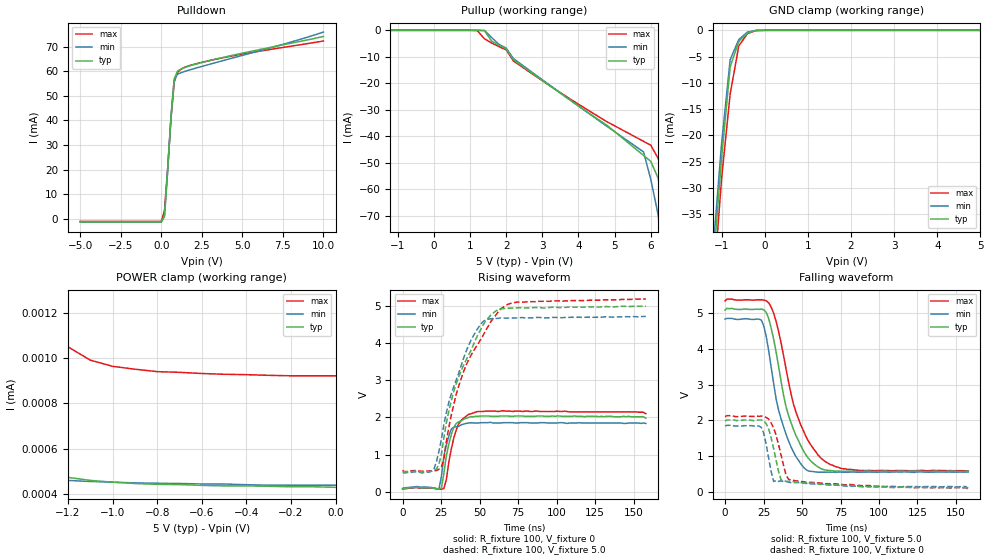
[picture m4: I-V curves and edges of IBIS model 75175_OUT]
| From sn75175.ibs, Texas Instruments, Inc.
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|   Model 75175_OUT
[Model]   75175_OUT
Model_type  3-state
Polarity   Non-Inverting
Enable   Active-Low
Vmeas = 1.3V
Cref = 15pf
Vref = 0V
| variable   typ   min   max
C_comp   3.716pf   3.575pf   4.006pf
[Temperature Range]   25   0   70
[Voltage Range]   5.0   4.75   5.25
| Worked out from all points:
|   slope of the pulldown table from 0 to 0.75 V, typ, clamps not added: 13.8 ohm
|   GND clamp passes 1 mA (typ) near -0.46 V on its own axis
|   rising waveform, R_fixture 100, V_fixture 0: 20-80 % time 5.45ns typ, 4.65ns min, 6.22ns max; typ from 0.094 V to 1.98 V
|   falling waveform, R_fixture 100, V_fixture 5.0: 20-80 % time 15.1ns typ, 13.2ns min, 17.4ns max; typ from 5.08 V to 0.587 V
|   rising waveform, R_fixture 100, V_fixture 5.0: 20-80 % time 20.8ns typ, 17.3ns min, 24ns max; typ from 0.548 V to 4.99 V
|   falling waveform, R_fixture 100, V_fixture 0: 20-80 % time 6.07ns typ, 4.76ns min, 7.27ns max; typ from 1.98 V to 0.096 V
[Pulldown]
|   Voltage   I(typ)   I(min   I(max)
-5V       -1.312mA   -1.5mA     -1.165mA
0V        -1.312mA   -1.5mA     -1.165mA
200mV     1.139mA    857.1uA    3.313mA
400mV     20.56mA    19.69mA    20.96mA
600mV     41.35mA    41.44mA    40.67mA
800mV     56.91mA    56.92mA    55.67mA
1V        60.09mA    58.87mA    59.6mA
1.2V      60.96mA    59.45mA    60.83mA
2V        62.77mA    61.12mA    62.88mA
3.8V      65.71mA    64.42mA    65.58mA
7.6V      70.99mA    71.26mA    69.9mA
10V       74.29mA    76.07mA    72.44mA
[Pullup]
|   Voltage   I(typ)   I(min)   I(max)
-5V       804.3nA    549.7nA    4.253uA
1.2V      674.3nA    480.3nA    -68.61uA
1.4V      -141.1uA   -2.019uA   -3.186mA
2V        -6.986mA   -6.679mA   -7.361mA
2.2V      -11.04mA   -10.61mA   -11.54mA
5.8V      -47.21mA   -45.89mA   -41.89mA
6V        -49.46mA   -56.21mA   -43.36mA
6.2V      -55.71mA   -69.38mA   -48.22mA
6.4V      -67.77mA   -92.52mA   -56.29mA
6.6V      -91.15mA   -115.7mA   -67.53mA
6.8V      -114.5mA   -138.8mA   -90.27mA
10V       -488.7mA   -509.1mA   -454.2mA
[GND Clamp]
|   Voltage   I(typ)   I(min)   I(max)
-5V       -487.7mA   -487.4mA   -481.7mA
-1.2V     -45.42mA   -42.15mA   -50.26mA
-1V       -24.41mA   -21.69mA   -28.36mA
-800mV    -6.951mA   -5.592mA   -12.12mA
-600mV    -2.132mA   -1.758mA   -2.98mA
-400mV    -465.2uA   -331.1uA   -618.5uA
-200mV    -20.85uA   -10.03uA   -50.72uA
0V        -253.2nA   159.5nA    -1.375uA
5V        429.3nA    439.1nA    909.8nA
[POWER Clamp]
|   Voltage   I(typ)   I(min)   I(max)
-5V       107.1uA    112.5uA    96.14uA
-1.7V     12.86uA    7.131uA    15.51uA
-1.6V     9.896uA    583.2nA    13.04uA
-1.5V     5.321uA    498.8nA    10.56uA
-1.4V     576.2nA    473.1nA    7.764uA
-1.3V     496nA      465.9nA    1.533uA
-1.2V     473.3nA    459.9nA    1.05uA
-1.1V     459.8nA    455.1nA    991.5nA
-1V       452.1nA    452.3nA    964.1nA
-800mV    442.5nA    447.3nA    940.7nA
-300mV    434nA      438.7nA    924.3nA
0V        429.3nA    438.7nA    922.3nA
[Ramp]
| variable   typ   min   max
dV/dt_r  1.100E+00/5.666E-09  1.100E+00/4.658E-09  1.200E+00/6.453E-09
dV/dt_f  2.700E+00/1.510E-08  2.600E+00/1.315E-08  2.900E+00/1.744E-09
R_load = 100
[Rising Waveform]
R_fixture = 100
V_fixture = 0
V_fixture_min = 0
V_fixture_max = 0
C_fixture = 0pf
L_fixture = 0nH
|   Time   V(typ)   V(min)   V(max)
0s        94mV       88mV       74mV
23.6ns    75.6mV     84.1mV     78.1mV
25.2ns    102mV      410mV      73.8mV
26.8ns    501mV      964mV      90.9mV
28.4ns    971mV      1.26V      330mV
31.6ns    1.54V      1.69V      1.15V
33.2ns    1.73V      1.74V      1.44V
36.4ns    1.88V      1.76V      1.83V
47.6ns    2.03V      1.85V      2.15V
158ns     1.98V      1.84V      2.1V
[Falling Waveform]
R_fixture = 100
V_fixture = 5.0
V_fixture_min = 4.75
V_fixture_max = 5.25
C_fixture = 0pf
L_fixture = 0nH
|   Time   V(typ)   V(min)   V(max)
0s        5.08V      4.83V      5.34V
22ns      5.1V       4.83V      5.37V
26.8ns    5.01V      4.33V      5.34V
31.6ns    4.26V      3.02V      4.99V
36.4ns    3.09V      2.04V      4.16V
44.4ns    1.75V      1.12V      2.46V
52.4ns    1.04V      628mV      1.56V
62ns      656mV      548mV      956mV
76.4ns    572mV      548mV      647mV
158ns     587mV      553mV      589mV
[Rising Waveform]
R_fixture = 100
V_fixture = 5.0
V_fixture_min = 4.75
V_fixture_max = 5.25
C_fixture = 0pf
L_fixture = 0nH
|   Time   V(typ)   V(min)   V(max)
0s        548.4mV    523.4mV    581mV
18.8ns    560.6mV    554.5mV    568mV
22ns      612.7mV    816.3mV    574mV
25.2ns    1.015V     1.416V     673mV
30ns      2.168V     2.405V     1.73V
36.4ns    3.083V     3.182V     2.84V
44.4ns    3.8V       4.075V     3.67V
54ns      4.597V     4.622V     4.34V
71.6ns    4.938V     4.671V     5.08V
158ns     4.989V     4.713V     5.18V
[Falling Waveform]
R_fixture = 100
V_fixture = 0
V_fixture_min = 0
V_fixture_max = 0
C_fixture = 0pf
L_fixture = 0nH
|   Time   V(typ)   V(min)   V(max)
0s        1.98V      1.84V      2.1V
23.6ns    2.01V      1.8V       2.12V
25.2ns    1.98V      1.63V      2.11V
28.4ns    1.75V      922mV      2.03V
31.6ns    1.2V       289mV      1.78V
34.8ns    561mV      291mV      1.31V
36.4ns    331mV      308mV      1.03V
39.6ns    292mV      290mV      472mV
42.8ns    282mV      258mV      326mV
158ns     96mV       99mV       75mV
